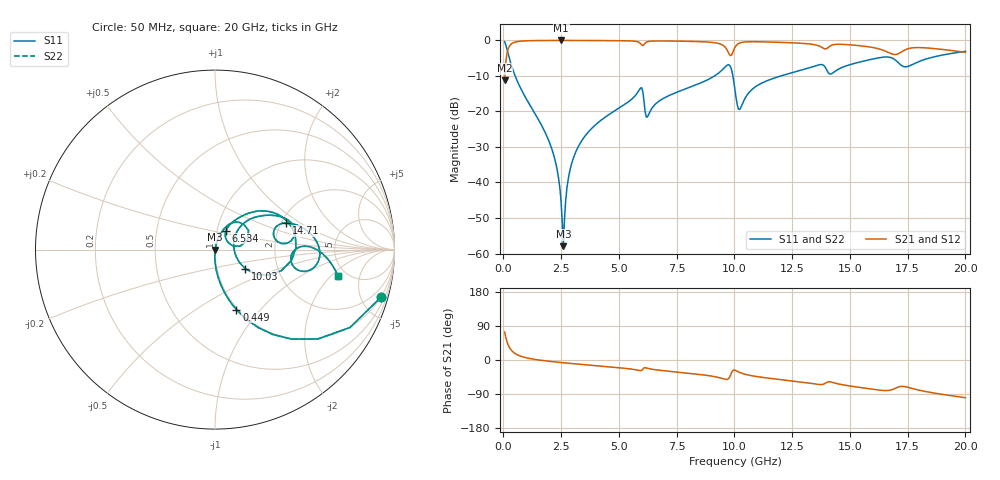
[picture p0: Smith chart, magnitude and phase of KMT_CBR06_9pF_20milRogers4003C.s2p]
! Data measured by Modelithics Inc. support@modelithics.com 813-866-6335
! KEMET CBR0603 9pF, Pad Width= 0.851mm, Pad Length= 0.64mm, Pad Gap= 0.62mm, 20mil Rogers 4003C substrate Data, January 2022
# hz S ma R 50
! 2 Port Network Data from SP1.SP block
! freq  magS11  angS11  magS21  angS21  magS12  angS12  magS22  angS22
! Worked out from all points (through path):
!   401 points, 50 MHz to 20 GHz, reference 50 ohm
!   highest |S21| = -0.01 dB at 2.494 GHz (marker M1); lowest = -11.2 dB at 50 MHz (marker M2)
!   group delay of S21, straight-line fit = 14.5 ps
!   lowest |S11| = -57.9 dB at 2.594 GHz (marker M3), VSWR 1.00, Z = 50.1 - j0.00477 ohm
!   |S11| at or under -10 dB: 506.5 MHz to 9.138 GHz (8.632 GHz wide, 179 % of centre); 9.932 GHz to 12.01 GHz (2.082 GHz wide, 19 % of centre)
!   |S22| runs from -57.9 to -0.3 dB; largest |S21 - S12| = 0
!   S11 on the Smith chart (normalised r, x): 50 MHz: 0.99, -6.96; 449 MHz: 0.99, -0.75; 6.534 GHz: 1.10, +0.24; 10.03 GHz: 1.37, -0.30; 14.71 GHz: 2.12, +0.77; 20 GHz: 4.21, -2.46
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5e7  0.9616 -16.1  0.2741 73.9  0.2741 73.9  0.9616 -16.1
4.49e8  0.3544 -70.4  0.9343 19.5  0.9343 19.5  0.3544 -70.4
2.045e9  0.03292 -91.9  0.9982 -3.9  0.9982 -3.9  0.03292 -91.9
2.34425e9  0.01396 -90.8  0.9986 -5.8  0.9986 -5.8  0.01396 -90.8
2.493875e9  0.00548 -83.6  0.9987 -6.7  0.9987 -6.7  0.00548 -83.6
2.593625e9  0.001269 -2.1  0.9986 -7.3  0.9986 -7.3  0.001269 -2.1
2.892875e9  0.01553 76.1  0.9984 -9.0  0.9984 -9.0  0.01553 76.1
3.391625e9  0.03885 76.1  0.9977 -11.7  0.9977 -11.7  0.03885 76.1
5.885375e9  0.2028 48.5  0.9322 -27.8  0.9322 -27.8  0.2028 48.5
6.2345e9  0.08384 41.4  0.9592 -21.7  0.9592 -21.7  0.08384 41.4
6.53375e9  0.1227 59.9  0.9819 -25.3  0.9819 -25.3  0.1227 59.9
6.73325e9  0.1396 60.3  0.983 -26.8  0.983 -26.8  0.1396 60.3
9.32675e9  0.3496 38.0  0.903 -46.4  0.903 -46.4  0.3496 38.0
9.72575e9  0.4541 9.6  0.691 -50.2  0.691 -50.2  0.4541 9.6
1.0025e10  0.2004 -32.2  0.8 -26.8  0.8 -26.8  0.2004 -32.2
1.02245e10  0.1064 10.5  0.9193 -32.6  0.9193 -32.6  0.1064 10.5
1.107238e10  0.2401 41.9  0.9561 -44.7  0.9561 -44.7  0.2401 41.9
1.336662e10  0.4231 24.7  0.8819 -62.0  0.8819 -62.0  0.4231 24.7
1.471325e10  0.4234 20.6  0.8786 -65.7  0.8786 -65.7  0.4234 20.6
1.670825e10  0.58 -6.2  0.6677 -80.0  0.6677 -80.0  0.58 -6.2
1.74065e10  0.4249 -5.9  0.741 -70.6  0.741 -70.6  0.4249 -5.9
2e10  0.7019 -12.2  0.6798 -99.6  0.6798 -99.6  0.7019 -12.2
